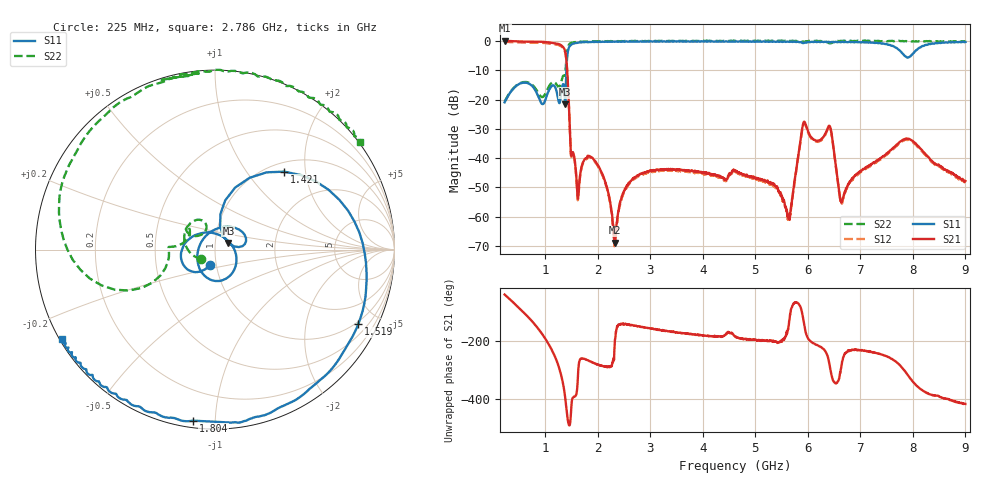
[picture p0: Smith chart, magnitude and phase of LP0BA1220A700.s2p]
!Agilent Technologies,E8358A,US41080443,A.07.50.56
!Agilent E8358A: A.07.50.56
!Date: Friday, July 08, 2016 13:29:47
!Correction: S11(Full 2 Port(1,2))
!S21(Full 2 Port(1,2))
!S12(Full 2 Port(1,2))
!S22(Full 2 Port(1,2))
!S2P File: Measurements: S11, S21, S12, S22:
# Hz S  dB  R 50
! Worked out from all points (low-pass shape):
!   1601 points, 225 MHz to 9 GHz, reference 50 ohm
!   highest |S21| = 0.14 dB at 225 MHz (marker M1); lowest = -68.9 dB at 2.32 GHz (marker M2)
!   |S21| within 3 dB of the highest: start of sweep to 1.368 GHz
!   lowest |S11| = -21.5 dB at 1.377 GHz (marker M3), VSWR 1.18, Z = 57.9 + j4.33 ohm
!   |S11| at or under -10 dB: start of sweep to 1.401 GHz
!   |S22| runs from -20.7 to 0.3 dB; largest |S21 - S12| = 0.041
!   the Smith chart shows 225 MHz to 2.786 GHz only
!   S11 on the Smith chart (normalised r, x): 225 MHz: 0.93, -0.16; 1.421 GHz: 1.17, +1.53; 1.519 GHz: 0.89, -3.89; 1.804 GHz: 0.04, -0.88; 2.786 GHz: 0.01, -0.27
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2.25e8  -20.89 -109.1  0.14 -37.3  -0.21 -37.0  -20.67 -145.5
6.089062e8  -14.15 -159.6  -0.13 -103.2  -0.48 -102.9  -13.95 135.5
9.434531e8  -21.50 65.0  -0.20 -175.2  -0.55 -175.1  -19.09 128.0
1.217672e9  -17.31 -129.2  -0.79 92.0  -1.13 92.1  -14.86 141.5
1.376719e9  -21.54 26.3  -3.33 -32.5  -3.67 -32.3  -11.32 -165.2
1.420594e9  -4.72 48.4  -11.30 -104.5  -11.61 -104.3  -2.91 -167.0
1.519312e9  -0.91 -27.6  -37.93 -37.0  -38.36 -37.3  -0.47 143.4
1.689328e9  -0.37 -70.6  -42.97 100.6  -43.35 100.8  -0.17 109.5
1.8045e9  -0.35 -97.2  -39.19 94.6  -39.42 94.9  -0.08 107.5
2.320031e9  -0.21 -134.4  -68.86 144.8  -67.51 135.0  0.06 64.0
2.786203e9  -0.11 -149.7  -45.70 -148.0  -46.05 -148.9  0.06 36.4
3.153656e9  -0.12 -158.1  -43.92 -159.9  -44.32 -159.1  0.11 19.5
4.6125e9  -0.13 -178.0  -44.12 177.2  -44.67 177.4  0.12 -22.3
5.632594e9  -0.20 162.6  -60.59 -147.2  -60.78 -142.1  0.19 -34.4
5.906812e9  -0.66 156.8  -28.50 -116.6  -28.78 -116.6  -0.14 -37.6
6.076828e9  -0.21 154.1  -33.01 156.6  -33.52 156.9  0.09 -37.4
6.422344e9  -0.37 145.7  -29.24 69.2  -29.47 69.2  -0.72 -40.7
6.647203e9  -0.21 140.2  -54.89 82.5  -55.50 83.1  0.07 -41.3
7.541156e9  -1.25 93.7  -37.80 105.3  -38.13 104.0  0.07 -54.0
7.831828e9  -4.78 10.8  -33.55 60.4  -33.91 60.5  -0.03 -59.0
8.018297e9  -3.94 -102.2  -34.48 16.1  -34.88 15.9  -0.10 -63.0
9e9  -0.25 160.9  -47.79 -57.5  -48.23 -58.6  -0.11 -86.5
